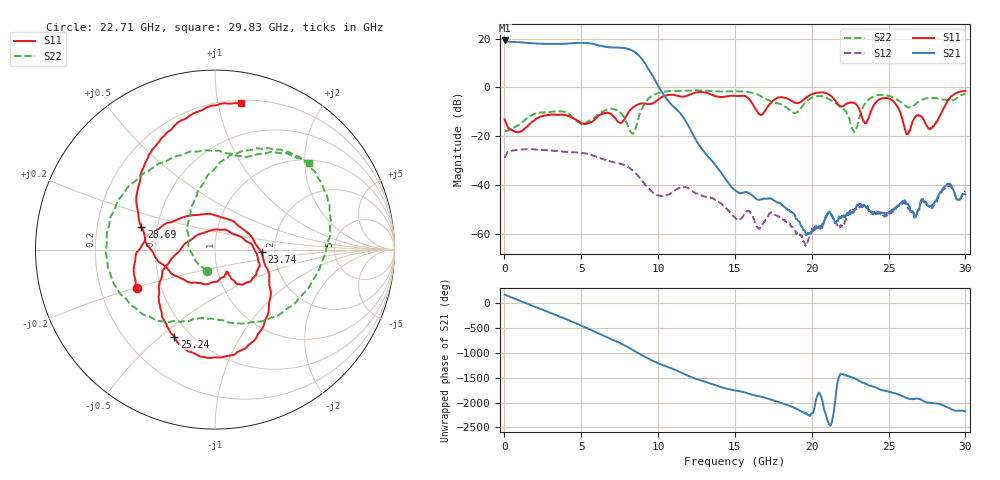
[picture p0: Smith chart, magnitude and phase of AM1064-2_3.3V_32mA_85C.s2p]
!Agilent	"Technologies,E8364B,MY43040894,A.07.50.67"
!Agilent	E8364B:	A.07.50.67
!Date:	"Wednesday,"	May	"01,"	2019	9:27:41
!Correction:	S11(Full	2	"Port(1,2))"
!S21(Full	2	"Port(1,2))"
!S12(Full	2	"Port(1,2))"
!S22(Full	2	"Port(1,2))"
!S2P	File:	Measurements:	"S11,"	"S21,"	"S12,"	S22:
#	Hz	S	dB	R	50
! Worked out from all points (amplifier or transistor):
!   1601 points, 10 MHz to 30 GHz, reference 50 ohm
!   highest |S21| = 19.2 dB at 10 MHz (marker M1)
!   |S21| within 3 dB of that: start of sweep to 7.47 GHz
!   unconditionally stable (mu >= 1): start of sweep to end of sweep
!   at 4.996 GHz: K = 1.49, MAG = 18.4 dB, |S12| = -26.9 dB
!   at 15.01 GHz: K = 5315.64, MAG = -34.7 dB, |S12| = -53.4 dB
!   at 30 GHz: K = 1414.15, MAG = -35.2 dB, |S12| = -42.5 dB
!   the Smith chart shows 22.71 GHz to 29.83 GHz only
!   S11 on the Smith chart (normalised r, x): 22.71 GHz: 0.36, -0.20; 23.74 GHz: 1.70, -0.05; 25.24 GHz: 0.41, -0.56; 28.69 GHz: 0.41, +0.13; 29.83 GHz: 0.22, +1.17
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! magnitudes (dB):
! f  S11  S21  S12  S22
! 10 MHz  -13.1  19.2  -28.9  -18.0
! 2.241 GHz  -12.4  17.9  -25.6  -10.5
! 5.015 GHz  -14.7  18.2  -26.9  -15.0
! 7.076 GHz  -11.7  16.3  -30.6  -8.9
! 8.351 GHz  -8.3  14.9  -34.1  -19.0
! 10.02 GHz  -5.0  0.4  -44.3  -2.3
! 11.84 GHz  -3.6  -14.3  -41.0  -1.4
! 15.01 GHz  -3.5  -42.2  -53.4  -1.7
! 16.69 GHz  -11.4  -45.9  -56.6  -3.7
! 17.42 GHz  -5.9  -45.9  -51.4  -6.1
! 18.88 GHz  -6.2  -52.2  -58.3  -10.5
! 20.01 GHz  -2.8  -57.9  -58.9  -4.2
! 22.71 GHz  -6.3  -51.3  -50.4  -17.8
! 23.74 GHz  -11.7  -50.5  -51.2  -4.8
! 25.01 GHz  -4.6  -51.4  -51.7  -3.5
! 25.24 GHz  -5.4  -50.4  -51.2  -4.1
! 26.23 GHz  -19.1  -47.9  -49.4  -8.2
! 26.78 GHz  -11.7  -53.1  -52.3  -6.9
! 27.73 GHz  -17.0  -48.4  -48.8  -4.4
! 28.69 GHz  -7.4  -40.4  -41.3  -5.1
! 29.83 GHz  -1.6  -43.7  -43.9  -3.0
! 30 GHz  -1.5  -43.9  -42.5  -2.8
